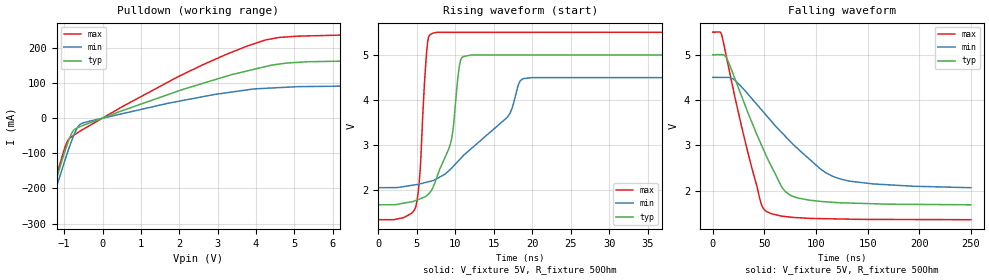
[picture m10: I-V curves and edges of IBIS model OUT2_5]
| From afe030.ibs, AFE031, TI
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|   OUT2 5V Model
[Model]  OUT2_5
Model_type   Open_drain
Polarity   Non-Inverting
Enable   Active-Low
Vmeas = 1.65
Vref = 1.65
Cref = 15pF
Rref = 50
|   typ   min   max
|   (nom PVT)   (slow PVT)   (fast PVT)
|   C_comp high output
C_comp   3.5320000e-12  2.7591950e-12   5.8438730e-12
|   typ   min   max
|   (nom PVT)   (Fast PVT)   (slow PVT)|   C_comp low output
|C_comp   2.0090270e-12  1.6664040e-12  2.3695140e-12
| Where   nom PVT is  Nominal Process, 5V, 52C
|   Fast PVT is Strong Process, 5.5V, -40C
|   Slow PVT is Weak Process, 4.5V, 150C
[Voltage Range]   5   4.5   5.5
[Temperature Range]   52   150   -40
[Pullup Reference]   5   4.5   5.5
[Pulldown Reference]   0   0   0
[Power Clamp Reference]   5   4.5   5.5
[GND Clamp Reference]   0   0   0
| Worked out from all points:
|   slope of the pulldown table from 0 to 0.75 V, typ, clamps not added: 24.9 ohm
|   falling waveform, V_fixture 5V, R_fixture 50Ohm: 20-80 % time 37.3ns typ, 62.2ns min, 25.8ns max; typ from 5 V to 1.68 V
|   rising waveform, V_fixture 5V, R_fixture 50Ohm: 20-80 % time 2.52ns typ, 7.87ns min, 796ps max; typ from 1.68 V to 5 V
[Pulldown]
|   Voltage   I(typ)   I(min)   I(max)
-5V       -1.708A    -1.64A     -1.866A
-1.683V   -355.1mA   -368.6mA   -358.7mA
-1.499V   -284.1mA   -301.9mA   -284.4mA
-1.17V    -162.2mA   -185.2mA   -152.3mA
-928.8mV  -77.67mA   -102.7mA   -68.38mA
-760.3mV  -35.5mA    -51.72mA   -49.75mA
-574.5mV  -23.88mA   -17.37mA   -36.39mA
1.95V     76.07mA    47.06mA    116.6mA
3.793V    134.6mA    80.55mA    205.8mA
4.598V    153.4mA    86.53mA    229.2mA
8.693V    166.9mA    93.92mA    242.6mA
10V       176mA      101.3mA    259.4mA
[Ramp]
R_load = 50
|   typ   min   max
dV/dt_r   1.98958/2.52615e-009   1.4631/7.86945e-009   2.48665/7.92654e-010
dV/dt_f   1.9895/3.73284e-008   1.4627/6.21071e-008   2.48663/2.58516e-008
[Falling Waveform]
V_fixture = 5V
V_fixture_min = 4.5V
V_fixture_max = 5.5V
R_fixture = 50Ohm
C_fixture = 0F
|   Time   V(typ)   V(min)   V(max)
0s        5V         4.5V       5.5V
8.604ns   5V         4.499V     5.442V
15.12ns   4.838V     4.498V     4.747V
33.35ns   3.763V     4.15V      2.9V
46.58ns   3.036V     3.8V       1.73V
51.32ns   2.792V     3.674V     1.545V
66.74ns   2.083V     3.282V     1.435V
74.84ns   1.899V     3.089V     1.413V
119.1ns   1.735V     2.288V     1.373V
250ns     1.684V     2.062V     1.356V
[Rising Waveform]
V_fixture = 5V
V_fixture_min = 4.5V
V_fixture_max = 5.5V
R_fixture = 50Ohm
C_fixture = 0F
|   Time   V(typ)   V(min)   V(max)
0s        1.684V     2.062V     1.356V
4.855ns   1.777V     2.127V     1.628V
5.438ns   1.817V     2.146V     2.426V
6.411ns   1.901V     2.188V     5.269V
7.63ns    2.3V       2.264V     5.492V
9.532ns   3.142V     2.496V     5.492V
10.7ns    4.876V     2.705V     5.492V
12.05ns   4.992V     2.92V      5.492V
19.93ns   4.993V     4.492V     5.493V
250ns     5V         4.5V       5.5V
